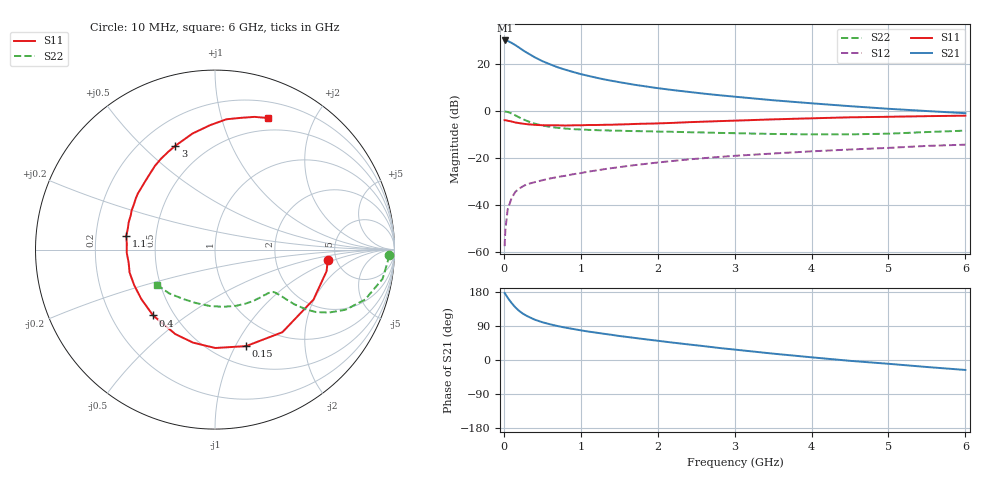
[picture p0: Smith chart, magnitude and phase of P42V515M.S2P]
! SIEMENS Small Signal Semiconductors
! BFP182
! Si NPN RF Bipolar Junction Transistor in SOT143
! VCE = 2.5 V  IC = 15 mA
! Common Emitter S-Parameters:  March  1996
# GHz  S  MA  R  50
!  f  S11  S21  S12  S22
! GHz  MAG  ANG  MAG  ANG  MAG  ANG  MAG  ANG
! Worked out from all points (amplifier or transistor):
!   36 points, 10 MHz to 6 GHz, reference 50 ohm
!   highest |S21| = 30.0 dB at 20 MHz (marker M1)
!   |S21| within 3 dB of that: start of sweep to 196.7 MHz
!   unconditionally stable (mu >= 1): 883.2 MHz to 5.346 GHz
!   at 250 MHz: K = 0.43, MSG = 29.0 dB, |S12| = -32.1 dB
!   at 1.4 GHz: K = 1.15, MAG = 16.3 dB, |S12| = -24.4 dB
!   at 6 GHz: K = 0.93, MSG = 6.7 dB, |S12| = -14.4 dB
!   S11 on the Smith chart (normalised r, x): 10 MHz: 4.24, -0.85; 150 MHz: 0.70, -1.10; 400 MHz: 0.38, -0.38; 1.1 GHz: 0.33, +0.07; 3 GHz: 0.34, +0.63; 6 GHz: 0.36, +1.42
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0.01  0.6308 -5.5  31.57 176.8  0.0013 88.7  0.9717 -1.9
0.02  0.6333 -10.9  31.79 174.0  0.0029 85.2  0.9647 -3.9
0.05  0.6154 -26.9  31.04 164.3  0.0079 81.7  0.9477 -9.9
0.1  0.594 -50.8  28.21 150.6  0.0137 67.8  0.8815 -18.4
0.15  0.565 -72.2  25.27 138.8  0.0188 61.3  0.8014 -24.7
0.2  0.5482 -89.9  22.32 129.4  0.022 56.3  0.7257 -28.9
0.25  0.5325 -103.3  19.55 122.0  0.0247 52.5  0.6625 -31.7
0.3  0.5202 -115.1  17.39 116.2  0.0272 50.1  0.6111 -33.2
0.4  0.5036 -133.2  13.97 106.6  0.0301 48.8  0.535 -34.6
0.5  0.4944 -146.1  11.53 99.7  0.0331 47.8  0.4877 -34.9
0.6  0.492 -156.2  9.87 94.3  0.0361 48.0  0.4566 -35.0
0.7  0.4928 -164.9  8.508 89.5  0.0389 48.6  0.4354 -35.2
0.9  0.4921 -178.0  6.765 81.9  0.0445 49.4  0.4079 -35.6
1.1  0.5001 171.2  5.576 75.0  0.0507 50.4  0.3937 -37.2
1.5  0.5131 154.8  4.099 63.4  0.063 50.4  0.3776 -41.6
1.8  0.5316 143.8  3.413 55.7  0.0726 49.9  0.3686 -45.9
2.2  0.5545 131.4  2.775 45.8  0.0855 47.6  0.3579 -52.7
3  0.6188 111.0  2.009 27.5  0.1099 41.6  0.3345 -69.5
3.5  0.659 100.9  1.686 16.8  0.1232 37.3  0.3217 -81.9
4.5  0.7289 85.0  1.26 -2.2  0.15 29.2  0.3159 -109.3
5.5  0.7717 73.4  0.992 -18.5  0.179 21.2  0.3535 -136.4
6  0.7903 68.0  0.892 -26.3  0.1902 16.2  0.3791 -149.1
